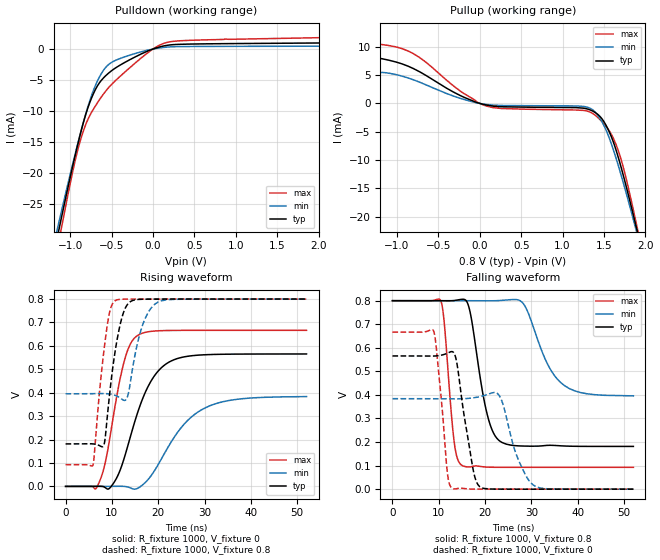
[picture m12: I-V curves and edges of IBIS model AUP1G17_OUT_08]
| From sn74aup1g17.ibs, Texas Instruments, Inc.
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[Model]   AUP1G17_OUT_08
Model_type  Output
Vref =   0
Rref =   1E6
Cref =   30p
Vmeas =   0.4
| variable   typ   min   max
C_comp   2.71pF   2.19pF   3.34pF
| C_pullup   2.77pF   2.20pF   3.34pF
| C_pulldown   2.64pF   2.19pF   3.08pF
[Temperature Range]   40   100   -40
| Ambient temperature   25   85   -40
[Voltage range]   0.8   0.8   0.8
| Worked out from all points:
|   slope of the pulldown table from 0 to 0.12 V, typ, clamps not added: 257 ohm
|   slope of the pullup table from 0 to 0.12 V, typ, clamps not added: 309 ohm
|   rising waveform, R_fixture 1000, V_fixture 0: 20-80 % time 6ns typ, 8.32ns min, 3.75ns max; typ from 0 V to 0.566 V
|   falling waveform, R_fixture 1000, V_fixture 0.8: 20-80 % time 3.19ns typ, 5.32ns min, 1.73ns max; typ from 0.8 V to 0.181 V
|   rising waveform, R_fixture 1000, V_fixture 0.8: 20-80 % time 2.57ns typ, 2.99ns min, 2.19ns max; typ from 0.181 V to 0.8 V
|   falling waveform, R_fixture 1000, V_fixture 0: 20-80 % time 2.64ns typ, 3.73ns min, 1.76ns max; typ from 0.566 V to 0 V
[Pulldown]
| AUP1G17_OUT_08
|   Voltage   I(typ)   I(min)   I(max)
-3.6V     -200.3mA   -184.7mA   -219.1mA
-1.155V   -30.43mA   -29.11mA   -32.45mA
-1.105V   -27.26mA   -26.22mA   -28.93mA
-940mV    -17.24mA   -17.01mA   -18.09mA
-865mV    -13.13mA   -13.1mA    -14.27mA
-745mV    -8.043mA   -7.657mA   -10.32mA
-630mV    -5.174mA   -4.128mA   -7.88mA
-470mV    -3.218mA   -1.946mA   -5.328mA
5mV       23.8uA     12.51uA    45.54uA
245mV     711.3uA    371.9uA    1.246mA
870mV     872.1uA    431.7uA    1.618mA
7.2V      1.459mA    578.6uA    3.138mA
[Pullup]
| AUP1G17_OUT_08
|   Voltage   I(typ)   I(min)   I(max)
-3.6V     2.784mA    339.2uA    9.474mA
-2.56V    3.921mA    663.8uA    11.14mA
-2.01V    6.261mA    1.269mA    13.37mA
-1.185V   7.906mA    5.477mA    10.41mA
-800mV    6.149mA    4.169mA    8.776mA
80mV      -287uA     -177.3uA   -461.9uA
1.285V    -921uA     -607uA     -1.305mA
1.455V    -2.355mA   -2.736mA   -2.902mA
1.625V    -7.333mA   -8.725mA   -6.56mA
1.74V     -13.09mA   -14.38mA   -11.68mA
1.905V    -22.78mA   -23.32mA   -22.23mA
7.2V      -396.8mA   -367.4mA   -431.7mA
[Ramp]
| AUP1G17_OUT_08
| variable   typ   min   max
dV/dt_r   0.35/6.07E-09   0.24/8.45E-09   0.41/3.81E-09
dV/dt_f   0.37/3.20E-09   0.25/5.35E-09   0.43/1.75E-09
R_load = 1000
[Rising Waveform]
| AUP1G17_OUT_08
R_fixture =   1000
C_fixture =   0
L_fixture =   0
V_fixture =   0
V_fixture_min = 0
V_fixture_max = 0
|   Time   V(typ)   V(min)   V(max)
0s        23.71nV    153.5nV    1.008nV
6.925ns   409.5uV    -5.943uV   3.275mV
8.625ns   -5.928mV   82.17uV    107.2mV
10.93ns   32.47mV    432.1uV    371.9mV
13.18ns   156mV      -1.451mV   569mV
15.54ns   314.5mV    -8.304mV   644.6mV
20.86ns   510mV      123.7mV    665.2mV
25.19ns   551.5mV    256.7mV    666.3mV
29.62ns   561.7mV    330.1mV    666.4mV
52ns      565.5mV    383.5mV    666.5mV
[Falling Waveform]
| AUP1G17_OUT_08
R_fixture =   1000
C_fixture =   0
L_fixture =   0
V_fixture =   0.8
V_fixture_min = 0.8
V_fixture_max = 0.8
|   Time   V(typ)   V(min)   V(max)
0s        800mV      800mV      800mV
10.45ns   799.8mV    800mV      798.3mV
13.31ns   800.7mV    800mV      203.5mV
14.91ns   805.8mV    800mV      102.1mV
16.55ns   769.4mV    799.9mV    94mV
20.18ns   339.3mV    799.6mV    93.94mV
22.97ns   207.1mV    800.5mV    92.79mV
28.24ns   183mV      787.6mV    92.73mV
37.14ns   183.2mV    439.4mV    92.72mV
52ns      181.5mV    396mV      92.72mV
[Rising Waveform]
| AUP1G17_OUT_08
R_fixture =   1000
C_fixture =   0
L_fixture =   0
V_fixture =   0.8
V_fixture_min = 0.8
V_fixture_max = 0.8
|   Time   V(typ)   V(min)   V(max)
0s        181.5mV    395.5mV    92.72mV
5.94ns    181.4mV    396mV      92.98mV
8.355ns   182.5mV    396.3mV    592mV
9.49ns    390.9mV    394.6mV    742.6mV
10.67ns   573.6mV    388.9mV    792.6mV
12.08ns   714.9mV    373.4mV    799.2mV
13.42ns   778.6mV    387.6mV    799.8mV
16.42ns   799.1mV    677mV      800mV
19.93ns   799.9mV    786.8mV    800mV
52ns      800mV      800mV      800mV
[Falling Waveform]
| AUP1G17_OUT_08
R_fixture =   1000
C_fixture =   0
L_fixture =   0
V_fixture =   0
V_fixture_min = 0
V_fixture_max = 0
|   Time   V(typ)   V(min)   V(max)
0s        565.5mV    384mV      666.5mV
8.915ns   565.1mV    383.8mV    669.4mV
11.85ns   577mV      383.5mV    70.2mV
12.86ns   583.9mV    383.4mV    4.201mV
17.49ns   75.76mV    387.8mV    303.8uV
18.89ns   10.01mV    392.7mV    51.34uV
23.12ns   160.4uV    395mV      827nV
26.87ns   10.37uV    139.6mV    325nV
30.66ns   839.8nV    14.17mV    -3.819nV
52ns      -855.4nV   -1.004uV   -297.7nV
